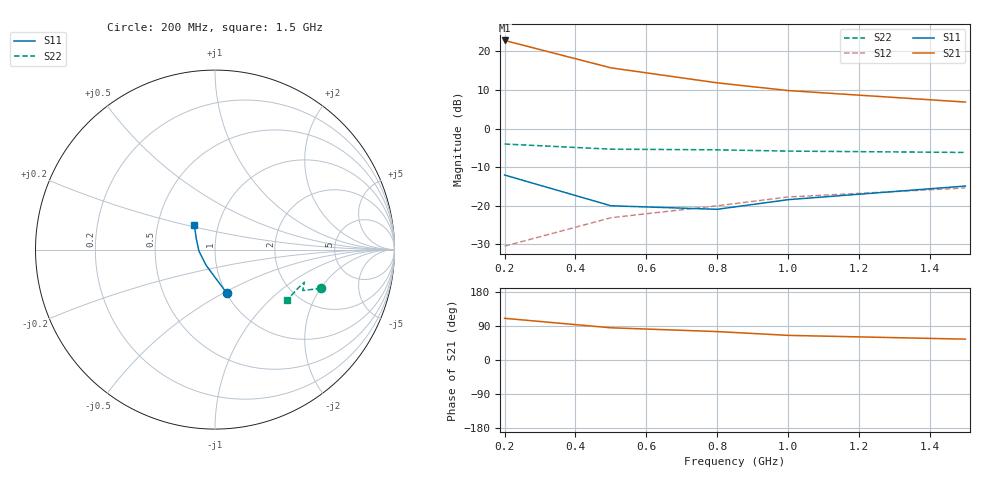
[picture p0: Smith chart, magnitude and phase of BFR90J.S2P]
!  BFR90J.S2P
!  BFR90
!  VCE=10V; IC=20mA
#  GHZ S MA R 50
!  S-PARAMETER DATA
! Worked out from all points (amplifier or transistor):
!   5 points, 200 MHz to 1.5 GHz, reference 50 ohm
!   highest |S21| = 22.8 dB at 200 MHz (marker M1)
!   |S21| within 3 dB of that: start of sweep to 326.9 MHz
!   unconditionally stable (mu >= 1): 490 MHz to end of sweep
!   at 200 MHz: K = 0.88, MSG = 26.6 dB, |S12| = -30.5 dB
!   at 800 MHz: K = 1.06, MAG = 14.4 dB, |S12| = -20.0 dB
!   at 1.5 GHz: K = 1.09, MAG = 9.3 dB, |S12| = -15.4 dB
0.2  0.25 -75.0  13.8 110.0  0.03 70.0  0.63 -20.0
0.5  0.1 -120.0  6.1 85.0  0.07 75.0  0.54 -25.0
0.8  0.09 -175.0  3.9 75.0  0.1 75.0  0.53 -20.0
1  0.12 150.0  3.1 65.0  0.13 75.0  0.51 -25.0
1.5  0.18 130.0  2.2 55.0  0.17 70.0  0.49 -35.0
